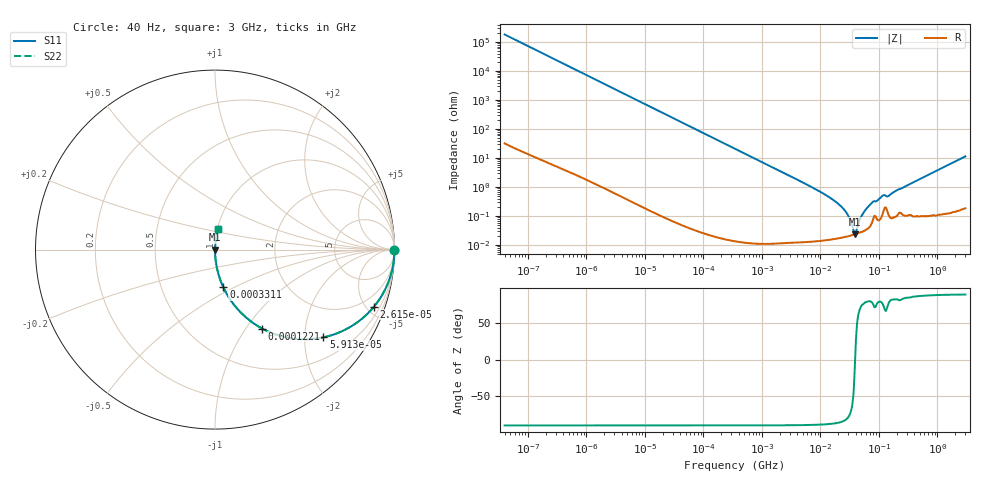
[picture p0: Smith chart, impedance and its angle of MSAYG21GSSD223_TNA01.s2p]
! MSAYG21GSSD223_TNA01  S-PARAMETER MODEL  ( General Type )
! Model Generated by TAIYO YUDEN Corporation (http://www.ty-top.com)
! Version 2.0
! TAIYO YUDEN Control No. 031016
! Copyright(c) 2003 TAIYO YUDEN CO.,LTD. All Rights Reserved.
! Product Description (link to TY-COMPAS)
! https://ds.yuden.co.jp/TYCOMPAS/or/detail?pn=MSAYG21GSSD223KTNA01&u=M
! Products Name : Multilayer Ceramic Capacitors
! Characteristics :
!  Capacitance : 0.022 uF , Rated Voltage : 35V
!  Case Size : 2.0 x 1.25 / 0.079 x 0.049 [mm/inch] , Thickness : 1.25 / 0.049 [mm/inch]
!  (Conditions: Temperature = 25 degC , DC Bias Current/Voltage = 0A / 0V)
! External Node Assignments :
!  1  o---| |---o  2
! GND o---------o GND
! Frequency Range : 40Hz  -  3GHz  [ 401 STEP ]
# MHz S RI R 50
! Freq[MHz].  S11 Real  S11 Imag  S21 Real  S21 Imag  S12 Real  S12 Imag  S22 Real  S22 Imag
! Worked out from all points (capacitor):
!   401 points, 40 Hz to 3 GHz, reference 50 ohm
!   read as one part in series: C = 21.8 nF near 44 Hz
!   lowest |Z| = 23.6 mohm at 38.65 MHz (marker M1)
!   series resonance near 39.1 MHz, so ESL is about 760 pH
!   S11 on the Smith chart (normalised r, x): 40 Hz: open; 26.14 kHz: 1.00, -5.58; 59.12 kHz: 1.00, -2.47; 122.1 kHz: 1.00, -1.20; 331.1 kHz: 1.00, -0.44; 3 GHz: 1.00, +0.23
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4e-05  1 -0.000548  3.96e-07 0.000548  3.96e-07 0.000548  1 -0.000548
0.000834  0.9999 -0.0114  0.000133 0.0114  0.000133 0.0114  0.9999 -0.0114
0.005113  0.9951 -0.0697  0.0049 0.0697  0.0049 0.0697  0.9951 -0.0697
0.017386  0.9463 -0.2253  0.0537 0.2253  0.0537 0.2253  0.9463 -0.2253
0.026145  0.8863 -0.3174  0.1137 0.3174  0.1137 0.3174  0.8863 -0.3174
0.059125  0.6039 -0.4889  0.3961 0.4889  0.3961 0.4889  0.6039 -0.4889
0.122117  0.2634 -0.4403  0.7366 0.4403  0.7366 0.4403  0.2634 -0.4403
0.331057  0.0465 -0.2102  0.9535 0.2102  0.9535 0.2102  0.0465 -0.2102
0.362475  0.0391 -0.1935  0.9609 0.1935  0.9609 0.1935  0.0391 -0.1935
1.178032  0.00393 -0.0617  0.9961 0.0617  0.9961 0.0617  0.00393 -0.0617
7.222098  0.000226 -0.00976  0.9998 0.00976  0.9998 0.00976  0.000226 -0.00976
14.91646  0.000172 -0.00416  0.9998 0.00416  0.9998 0.00416  0.000172 -0.00416
22.43131  0.000182 -0.00217  0.9998 0.00217  0.9998 0.00217  0.000182 -0.00217
29.4429  0.000201 -0.00106  0.9998 0.00106  0.9998 0.00106  0.000201 -0.00106
36.93337  0.000227 -0.00022  0.9998 0.00022  0.9998 0.00022  0.000227 -0.00022
38.64618  0.000232 -4.33e-05  0.9998 4.33e-05  0.9998 4.33e-05  0.000232 -4.33e-05
42.31378  0.000251 0.000304  0.9997 -0.000304  0.9997 -0.000304  0.000251 0.000304
53.07868  0.000298 0.00116  0.9997 -0.00116  0.9997 -0.00116  0.000298 0.00116
72.90103  0.0005 0.00263  0.9995 -0.00263  0.9995 -0.00263  0.0005 0.00263
114.7124  0.00116 0.00482  0.9988 -0.00482  0.9988 -0.00482  0.00116 0.00482
150.5692  0.000996 0.00508  0.999 -0.00508  0.999 -0.00508  0.000996 0.00508
3000  0.0147 0.1125  0.9853 -0.1125  0.9853 -0.1125  0.0147 0.1125
